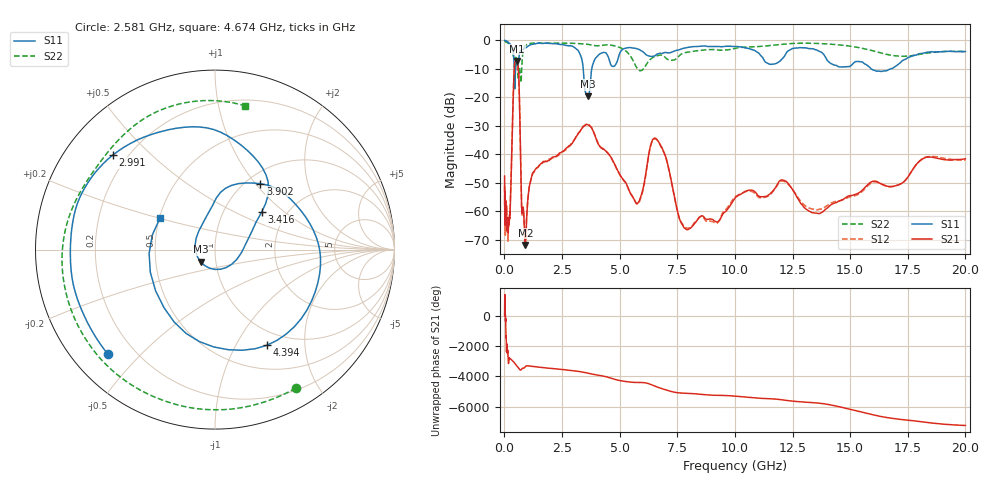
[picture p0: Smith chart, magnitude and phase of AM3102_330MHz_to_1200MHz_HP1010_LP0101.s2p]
! Date/Time: Tue, Sep 11, 2018 5:19 PM
! Network Analyzer: Agilent Technologies E8362B Rev: A.07.50.63
! Sweep from 0.010 to 20.000 GHz, 1601 Points, Sweep Type: LOG
! Power Supply: 4.949 V, 0.001 A
# Hz S DB R 50
!freq MagS11 AngS11 MagS21 AngS21 MagS12 AngS12 MagS22 AngS22
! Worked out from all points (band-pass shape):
!   1601 points, 10 MHz to 20 GHz, reference 50 ohm
!   highest |S21| = -7.19 dB at 551.2 MHz (marker M1); lowest = -71.8 dB at 912 MHz (marker M2)
!   |S21| within 3 dB of the highest: 425.8 MHz to 608.8 MHz (183 MHz wide, 35.4 % of centre)
!   lowest |S11| = -19.6 dB at 3.617 GHz (marker M3), VSWR 1.23, Z = 42.2 - j5.73 ohm
!   |S11| at or under -10 dB: 425.2 MHz to 479.2 MHz (54.01 MHz wide, 11.9 % of centre); 3.421 GHz to 3.791 GHz (369.8 MHz wide, 10.3 % of centre); 15.91 GHz to 16.77 GHz (853 MHz wide, 5.22 % of centre)
!   |S22| runs from -14.8 to -0.2 dB; largest |S21 - S12| = 0.0063
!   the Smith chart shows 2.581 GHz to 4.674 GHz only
!   S11 on the Smith chart (normalised r, x): 2.581 GHz: 0.11, -0.40; 2.991 GHz: 0.15, +0.39; 3.416 GHz: 1.50, +0.71; 3.902 GHz: 1.16, +1.06; 4.394 GHz: 0.80, -1.35; 4.674 GHz: 0.50, +0.20
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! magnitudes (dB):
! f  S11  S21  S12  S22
! 10 MHz  0.0  -47.6  -53.0  -0.2
! 35.55 MHz  0.0  -61.9  -64.2  -0.3
! 126.4 MHz  -0.4  -64.1  -63.9  -0.8
! 250.5 MHz  -1.3  -59.2  -58.7  -1.5
! 447.2 MHz  -16.9  -8.0  -8.0  -6.7
! 551.2 MHz  -7.9  -7.2  -7.2  -8.5
! 635.6 MHz  -5.7  -15.5  -15.5  -10.2
! 754.2 MHz  -3.2  -59.1  -60.1  -9.6
! 912 MHz  -2.7  -71.8  -71.8  -1.8
! 1.103 GHz  -1.6  -50.5  -50.5  -1.1
! 1.59 GHz  -1.0  -43.2  -43.3  -0.9
! 2.581 GHz  -1.6  -38.8  -38.8  -1.0
! 2.991 GHz  -2.2  -35.4  -35.4  -1.0
! 3.416 GHz  -9.5  -30.2  -30.5  -1.2
! 3.617 GHz  -19.6  -29.6  -29.4  -1.4
! 3.902 GHz  -7.0  -32.8  -32.7  -1.8
! 4.394 GHz  -4.3  -38.8  -38.7  -1.6
! 4.674 GHz  -9.0  -41.8  -41.9  -1.7
! 5.652 GHz  -2.7  -56.2  -56.2  -8.2
! 6.549 GHz  -5.3  -34.3  -34.6  -5.6
! 7.958 GHz  -2.4  -66.5  -66.0  -4.1
! 20 GHz  -3.9  -41.6  -42.1  -3.8
